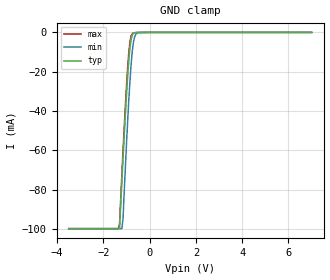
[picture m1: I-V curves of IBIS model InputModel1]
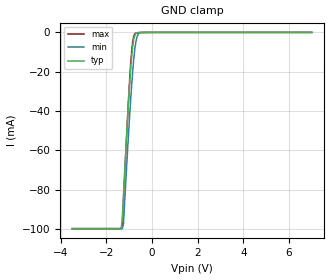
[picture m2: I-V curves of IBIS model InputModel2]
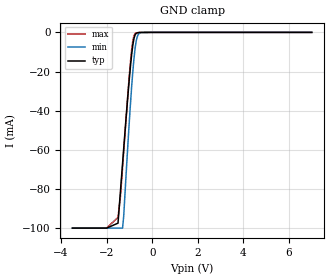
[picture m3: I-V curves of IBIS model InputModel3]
[IBIS Ver]   2.1
[File name]   e_400cv3.ibs   | e= TSOP, f400cv= abbr chip name, 3= 3.3V Vcc
[File Rev]   2.00
[Date]   13-March-1996
[Source]   File generated from lab measurements at Intel Corporation
[Notes]   Rev 2.00 All data was replaced by actual measurements
   performed in a lab.
[Disclaimer] INTEL DEVELOPER'S SOFTWARE LICENSE AGREEMENT
| BY USING THIS SOFTWARE, YOU ARE AGREEING TO BE BOUND
| BY THE TERMS OF THIS AGREEMENT.  DO NOT USE THE SOFTWARE
| UNTIL YOU HAVE CAREFULLY READ AND AGREED TO THE FOLLOWING
| TERMS AND CONDITIONS.  IF YOU DO NOT AGREE TO THE TERMS
| OF THIS AGREEMENT, PROMPTLY RETURN THE SOFTWARE PACKAGE
| AND ANY ACCOMPANYING ITEMS.
| IF YOU USE THIS SOFTWARE, YOU WILL BE BOUND BY THE TERMS
| OF THIS AGREEMENT
| LICENSE: Intel Corporation ("Intel") grants you the non-exclusive right
| to use the enclosed software program ("Software").  You will not use,
| copy, modify, rent, sell or transfer the Software or any portion
| thereof, except as provided in this Agreement.
| System OEM Developers may:
| 1.   Copy the Software for support, backup or archival purposes;
| 2.   Install, use, or distribute Intel owned Software in object code
|   only;
| 3.   Modify and/or use Software source code that Intel directly makes
|   available to you as an OEM Developer;
| 4.   Install, use, modify, distribute, and/or make or have made
|   derivatives ("Derivatives") of Intel owned Software under the
|   terms and conditions in this Agreement, ONLY if you are a System
|   OEM Developer and NOT an end-user.
| RESTRICTIONS:
| YOU WILL NOT:
| 1.   Copy the Software, in whole or in part, except as provided for
|   in this Agreement;
| 2.   Decompile or reverse engineer any Software provided in object
|   code format;
| 3.   Distribute any Software or Derivative code to any end-users,
|   unless approved by Intel in a prior writing.
| TRANSFER: You may transfer the Software to another OEM
| Developer if the receiving party agrees to the terms of this
| Agreement at the sole risk of any receiving party.
| OWNERSHIP AND COPYRIGHT OF SOFTWARE:
| Title to the Software and all copies thereof remain with Intel
| or its vendors.  The Software is copyrighted and is protected by
| United States and international copyright laws.  You will not
| remove the copyright notice from the Software.  You agree to
| prevent any unauthorized copying of the Software.
| DERIVATIVE WORK: OEM Developers that make or have made
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[Copyright]   Copyright 1996, Intel Corporation, All Rights Reserved
[Component]   E28F400CV   | 48-lead TSOP package, 28F400CV
[Manufacturer]  Intel   | Boot Block (tm)
|   | operating in 3.3V Vcc range
[Package]
R_pkg   48.0m   41.0m   54.0m
L_pkg   4.92nH   4.44nH   5.39nH
C_pkg   0.48pF   0.45pF   0.50pF
|*****************************Pin Definitions*****************************
[Pin]   signal_name   model_name   R_pin   L_pin   C_pin
 1   A15   InputModel3
 2   A14   InputModel3
 3   A13   InputModel3
 4   A12   InputModel3
 5   A11   InputModel3
 6   A10   InputModel3
 7   A09   InputModel3
 8   A08   InputModel3
 9   NC   InputModel4
10   NC   InputModel4
11   WE#   InputModel1
12   RP#   InputModel1
13   VPP   POWER
14   WP#   InputModel1
15   NC   InputModel4
16   NC   InputModel3
17   A17   InputModel3
18   A07   InputModel3
19   A06   InputModel3
20   A05   InputModel3
21   A04   InputModel3
22   A03   InputModel3
23   A02   InputModel3
24   A01   InputModel3
25   A00   InputModel2
26   CE#   InputModel1
27   GND   GND
28   OE#   InputModel1
29   DQ0   InputOutput
30   DQ8   InputOutput
31   DQ1   InputOutput
32   DQ9   InputOutput
33   DQ2   InputOutput
34   DQ10   InputOutput
35   DQ3   InputOutput
36   DQ11   InputOutput
37   VCC   POWER
38   DQ4   InputOutput
39   DQ12   InputOutput
40   DQ5   InputOutput
41   DQ13   InputOutput
42   DQ6   InputOutput
43   DQ14   InputOutput
44   DQ7   InputOutput
45   DQ15   InputOutput
46   GND   GND
47   BYTE#   InputModel2
48   A16   InputModel2
|***********************Input Model 4******************************
[Model]   InputModel4
Model_type   Input
|   Model for all NC pins, excluding NC pin #16.
Vinl = 0.8V
Vinh = 2.0V
|Variable   Typ   Min   Max
C_comp   5.61p   NA   7.6p
[Voltage Range]   3.3V   3.0V   3.6V
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| Models and submodels in the file (5): InputModel1 (Input), InputModel2 (Input), InputModel3 (Input), InputModel4 (Input), InputOutput (I/O)
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|*********************Input Model 1************************************
[Model]   InputModel1
Model_type   Input
|   Model for WE#, WP#, RP#, OE# & CE#.
Vinl = 0.8V
Vinh = 2.0V
|Variable   Typ   Min   Max
C_comp   5.61p   NA   7.6p
[Voltage Range]   3.3V   3.0V   3.6V
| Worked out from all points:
|   GND clamp passes 1 mA (typ) near -0.73 V on its own axis
[GND_clamp]
|Voltage  I(typ)   I(min)   I(max)
-3.5V     -99.85mA   -99.85mA   -99.85mA
-1.35V    -99.85mA   -99.85mA   -99.85mA
-1.3V     -99.26mA   -99.85mA   -97.14mA
-1.2V     -75.18mA   -99.85mA   -72.14mA
-1.15V    -63.89mA   -94.76mA   -60.07mA
-1V       -31.6mA    -56.54mA   -27.07mA
-900mV    -14.05mA   -34.26mA   -10.17mA
-850mV    -7.687mA   -24.68mA   -4.745mA
-750mV    -1.284mA   -9.549mA   -630.3uA
-650mV    -225.8uA   -2.279mA   -169.1uA
-500mV    -29.1uA    -152uA     -20.31uA
7V        0A         0A         0A
[Power_clamp]
| Input buffer circuits of this product do not intrinsically
| require a [Power_clamp] definition.  This zero current
| [Power_clamp] table is provided for the compatibility with
| some IBIS parsers.
|Voltage  I(typ)   I(min)   I(max)
-3.3V     0A         0A         0A
0V        0A         0A         0A
3.3V      0A         0A         0A
7V        0A         0A         0A
|*********************Input Model 2******************************
[Model]   InputModel2
Model_type   Input
|   Model for A[0], A[16] & BYTE# pins.
Vinl = 0.8V
Vinh = 2.0V
|Variable   Typ   Min   Max
C_comp   5.61p   NA   7.6p
[Voltage Range]   3.3V   3.0V   3.6V
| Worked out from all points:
|   GND clamp passes 1 mA (typ) near -0.73 V on its own axis
[GND_clamp]
|Voltage  I(typ)   I(min)   I(max)
-3.5V     -99.85mA   -99.83mA   -99.85mA
-1.35V    -99.85mA   -99.83mA   -99.85mA
-1.3V     -94.37mA   -99.83mA   -98.64mA
-1.25V    -82.89mA   -97.51mA   -85.83mA
-1.1V     -50.15mA   -66.04mA   -49.42mA
-950mV    -21.04mA   -36.93mA   -18.24mA
-900mV    -13.36mA   -28.31mA   -10.32mA
-850mV    -7.565mA   -20.57mA   -4.846mA
-750mV    -1.296mA   -8.199mA   -639.8uA
-650mV    -228.2uA   -2.043mA   -174.9uA
-500mV    -30.35uA   -138.9uA   -20.97uA
7V        0A         0A         0A
[Power_clamp]
| Input buffer circuits of this product do not intrinsically
| require a [Power_clamp] definition.  This zero current
| [Power_clamp] table is provided for the compatibility with
| some IBIS parsers.
|Voltage  I(typ)   I(min)   I(max)
-3.3V     0A         0A         0A
0V        0A         0A         0A
3.3V      0A         0A         0A
7V        0A         0A         0A
|***********************Input Model 3******************************
[Model]   InputModel3
Model_type   Input
|   Model for A[15:1], A[17] & NC pin #16.
Vinl = 0.8V
Vinh = 2.0V
|Variable   Typ   Min   Max
C_comp   5.61p   NA   7.6p
[Voltage Range]   3.3V   3.0V   3.6V
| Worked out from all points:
|   GND clamp passes 1 mA (typ) near -0.73 V on its own axis
[GND_clamp]
|Voltage  I(typ)   I(min)   I(max)
-3.5V     -99.85mA   -99.85mA   -99.84mA
-2V       -99.85mA   -99.85mA   -99.84mA
-1.5V     -97.31mA   -99.85mA   -94.31mA
-1.4V     -82.07mA   -99.85mA   -84.51mA
-1.3V     -66.84mA   -99.85mA   -68.9mA
-1.25V    -59.17mA   -93.69mA   -60.87mA
-950mV    -16.82mA   -35.79mA   -14.52mA
-850mV    -6.51mA    -20.05mA   -4.331mA
-750mV    -1.251mA   -8.08mA    -628.9uA
-650mV    -222.2uA   -2.03mA    -171.1uA
-500mV    -30.37uA   -137.4uA   -20.58uA
7V        0A         0A         0A
[Power_clamp]
| Input buffer circuits of this product do not intrinsically
| require a [Power_clamp] definition.  This zero current
| [Power_clamp] table is provided for the compatibility with
| some IBIS parsers.
|Voltage  I(typ)   I(min)   I(max)
-3.3V     0A         0A         0A
0V        0A         0A         0A
3.3V      0A         0A         0A
7V        0A         0A         0A
